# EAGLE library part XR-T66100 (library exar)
Caller ID RECEIVER
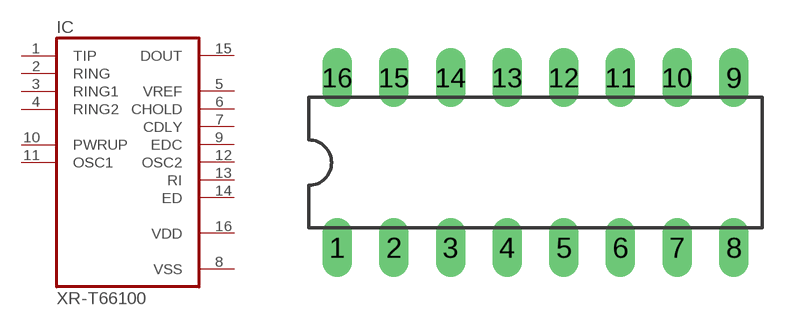
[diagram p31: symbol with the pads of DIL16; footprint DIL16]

Designator prefix IC

## XR-T66100 (OC_FARNELL: unknown; OC_NEWARK: unknown)  [DIL16]
1  TIP  in
2  RING  in
3  RING1  in
4  RING2  in
5  VREF  out
6  CHOLD  out
7  CDLY  out
8  VSS  pwr
9  EDC  out
10  PWRUP  in
11  OSC1  in
12  OSC2  out
13  RI  out
14  ED  out
15  DOUT  out
16  VDD  pwr

## Footprint DIL16 (pad centres in mm)
Dual In Line Package
drill 0.813 long: 1 -8.89,-3.81; 2 -6.35,-3.81; 3 -3.81,-3.81; 4 -1.27,-3.81; 5 1.27,-3.81; 6 3.81,-3.81; 7 6.35,-3.81; 8 8.89,-3.81; 9 8.89,3.81; 10 6.35,3.81; 11 3.81,3.81; 12 1.27,3.81; 13 -1.27,3.81; 14 -3.81,3.81; 15 -6.35,3.81; 16 -8.89,3.81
